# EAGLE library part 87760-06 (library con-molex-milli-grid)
HEADER
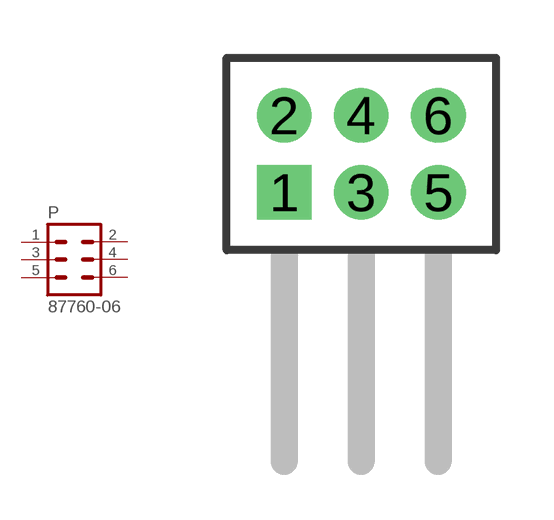
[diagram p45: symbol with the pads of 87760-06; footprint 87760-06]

Designator prefix P

## 87760-06  [87760-06]
1  1  pas
2  2  pas
3  3  pas
4  4  pas
5  5  pas
6  6  pas

## Footprint 87760-06 (pad centres in mm)
HEADER Dual Row, Right Angle
drill 0.914 square: 1 -2,-1
drill 0.914: 2 -2,1; 3 0,-1; 4 0,1; 5 2,-1; 6 2,1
